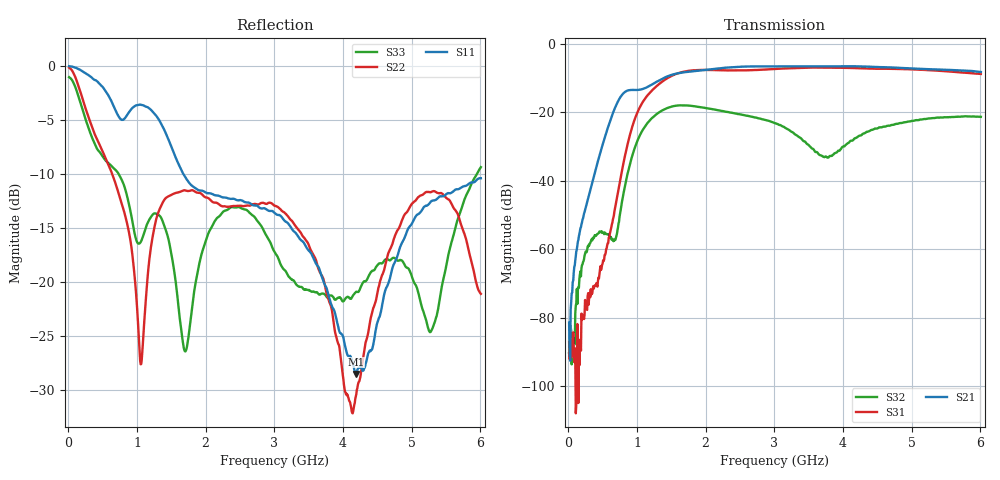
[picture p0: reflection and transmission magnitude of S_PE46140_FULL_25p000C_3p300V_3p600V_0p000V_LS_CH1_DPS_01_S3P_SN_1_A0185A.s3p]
! Device ID: PE46140_FULL
! File Path: z:\PE46140\MajorStates\25p000C\3p300\LS_CH1_DPS_01\PE46140_FULL_25p000C_3p300V_3p600V_0p000V_LS_CH1_DPS_01_S3P_SN_1_A0185A.s3p
! Serial: 1
! Lot: A0185A
! Temp: 25.000C
! VDD: 3.300
! VSS: 0.000
! Control_Hi: 3.600
! Control_Lo: 0.000
! Logic State: LS_CH1_DPS_01
! Port 1: RFIN
! Port 2: RFOUT1
! Port 3: RFOUT2
! ThroughPath:1-2
! IDD: 0.0003111428
! ISS: -1.769e-007
! Comment:
#  Hz  S  RI  R  50
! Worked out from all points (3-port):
!   801 points, 10 MHz to 6.01 GHz, reference 50 ohm
!   strongest paths, dB at 10 MHz, 1.51 GHz, 3.01 GHz, 4.51 GHz, 6.01 GHz:
!     S21: -81.5, -9.1, -6.7, -6.9, -8.3
!     S31: -87.1, -9.4, -7.4, -7.4, -8.9
!     S32: -90.3, -18.4, -23.2, -24.7, -21.4
!   lowest |S11| = -28.5 dB at 4.188 GHz (marker M1), VSWR 1.08, Z = 46.9 + j1.97 ohm
!   |S11| at or under -10 dB: 1.672 GHz to end of sweep
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1e7  0.9922 -0.0708  8.33e-05 2.12e-05  2.96e-05 -8.95e-06
     6.28e-05 5.62e-05  0.9748 -0.0927  -1.56e-05 3.99e-05
     -2.85e-05 -3.38e-05  -1.5e-05 2.65e-05  0.8809 -0.083
3.25e8  -0.2977 -0.8374  -0.00756 0.00122  -8.1e-05 0.000192
        -0.00755 0.00115  -0.4214 -0.3389  -0.000413 0.00123
        -6.59e-05 0.00025  -0.000417 0.00121  -0.3784 -0.2988
7.825e8  -0.5573 -0.0653  -0.000508 0.1786  0.0143 -0.00185
         -0.000532 0.1788  0.0658 0.2167  -0.00129 0.00485
         0.0141 -0.00178  -0.00129 0.00489  0.0761 0.2834
1.06e9  -0.6365 0.1717  0.1965 0.0822  -0.0702 -0.1062
        0.1968 0.083  -0.00776 -0.0409  0.0155 -0.0474
        -0.0701 -0.1065  0.0154 -0.0473  0.1114 0.1069
1.3825e9  -0.3375 0.3897  0.2874 -0.12  -0.1762 0.2239
          0.2877 -0.1198  -0.0344 0.2327  -0.0562 0.0915
          -0.1767 0.2241  -0.0563 0.0916  0.1741 -0.068
1.96e9  -0.1312 0.228  -0.145 -0.3816  0.4087 -0.0446
        -0.1451 -0.3818  0.2188 0.1232  0.0431 -0.1078
        0.4089 -0.0444  0.0433 -0.1076  0.0451 0.1337
3.01e9  0.00843 0.2074  -0.2 0.4175  -0.3686 -0.2106
        -0.2008 0.4174  0.204 -0.0943  0.0398 0.056
        -0.369 -0.2111  0.0399 0.0561  0.1267 -0.05
4.1875e9  -0.0311 0.021  0.4369 -0.1579  0.121 0.4199
          0.4371 -0.1576  0.0289 0.0059  0.019 0.0373
          0.1214 0.4199  0.0191 0.0371  0.0874 -0.0197
5.11e9  -0.1395 -0.1525  -0.2491 -0.3474  0.3791 -0.1687
        -0.2486 -0.348  0.2473 0.0199  -0.0595 -0.0484
        0.3792 -0.1684  -0.0591 -0.0483  0.0694 -0.0505
6.01e9  -0.2518 -0.1656  -0.2209 0.3133  -0.1638 -0.3194
        -0.2211 0.313  0.087 -0.0129  0.0357 0.077
        -0.165 -0.3198  0.0362 0.077  0.3168 0.1212
